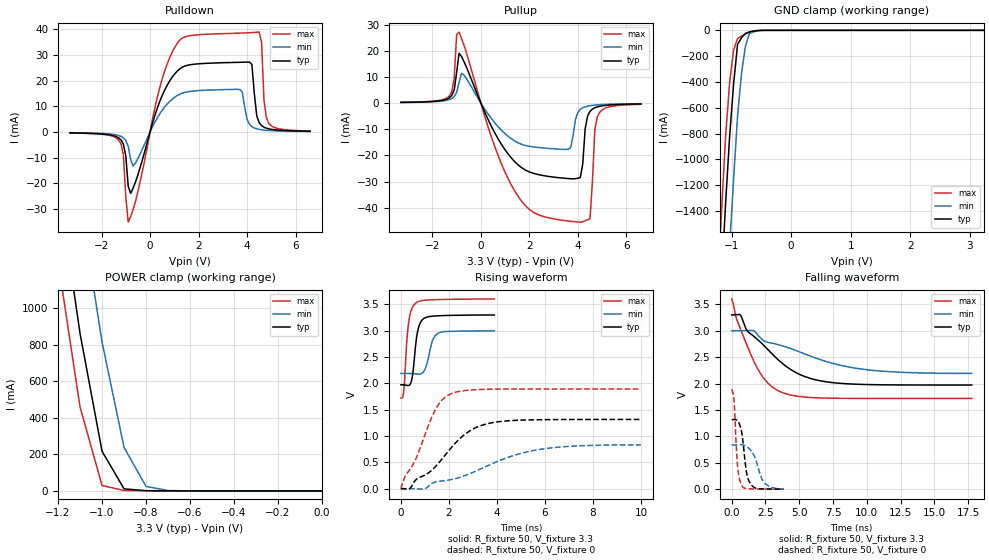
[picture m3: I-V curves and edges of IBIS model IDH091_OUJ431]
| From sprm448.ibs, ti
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|BUFFER IN NORMAL MODE WITHOUT PULLUP/PULLDOWN
|   Model Cell IDH091_OUJ431
|IDH091_OUJ431
[Model]   IDH091_OUJ431
Model_type   I/O
Polarity   Non-Inverting
Enable   Active-Low
Vinl =  0.8v
Vinh =  2v
Cref =  15.0000pF
Rref =  100.0000M
Vref =  0V
Vmeas =  1.65
C_comp   2.2553p   1.8929p   2.9061p
[Model Spec]
Vinl   0.8v   0.8v   0.8v
Vinh   2v   2v   2v
[Temperature Range]   25   125   -40
[Voltage Range]   3.3   3   3.6
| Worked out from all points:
|   slope of the pulldown table from 0 to 0.495 V, typ, clamps not added: 35.1 ohm
|   slope of the pullup table from 0 to 0.495 V, typ, clamps not added: 49.5 ohm
|   GND clamp passes 1 mA (typ) near -0.52 V on its own axis
|   POWER clamp passes 1 mA (typ) near -0.78 V on its own axis
|   rising waveform, R_fixture 50, V_fixture 3.3: 20-80 % time 211ps typ, 268ps min, 187ps max; typ from 1.97 V to 3.3 V
|   rising waveform, R_fixture 50, V_fixture 0: 20-80 % time 1.71ns typ, 2.93ns min, 1.06ns max; typ from 0 V to 1.31 V
|   falling waveform, R_fixture 50, V_fixture 3.3: 20-80 % time 3.49ns typ, 5.67ns min, 2.03ns max; typ from 3.3 V to 1.97 V
|   falling waveform, R_fixture 50, V_fixture 0: 20-80 % time 386ps typ, 697ps min, 250ps max; typ from 1.31 V to 0.002 V
[POWER_clamp]
|   voltage   I(typ)   I(min)   I(max)
-3.3V     22.03A     22.67A     21.68A
-1.2V     1.688A     2.438A     1.256A
-1.167V   1.413A     2.154A     990.6mA
-1.133V   1.137A     1.87A      725mA
-1.1V     861.3mA    1.585A     459.4mA
-1.033V   431.8mA    1.071A     173mA
-1V       217.1mA    814.3mA    29.74mA
-900mV    11.3mA     237.8mA    2.297mA
-800mV    1.149mA    24.8mA     1.228mA
-700mV    480.7uA    1.953mA    593.6uA
-11.55fV  74.41pA    10.75nA    861.5fA
[Pulldown]
|   voltage   I(typ)   I(min)   I(max)
-3.3V     -331.4uA   -255uA     -371.5uA
-1.3V     -2.223mA   -1.332mA   -3.045mA
-1.1V     -4.741mA   -2.234mA   -8.773mA
-900mV    -21.12mA   -5.605mA   -35.11mA
-700mV    -21.88mA   -13.27mA   -30.21mA
1.1V      23.53mA    14.08mA    34.28mA
3.7V      27.17mA    16.59mA    38.53mA
4.1V      27.25mA    2.984mA    38.69mA
4.5V      3.644mA    1.04mA     38.93mA
4.7V      1.881mA    774.1uA    12.24mA
4.9V      1.25mA     615uA      3.388mA
6.6V      316.3uA    220.9uA    418.1uA
[Pullup]
|   voltage   I(typ)   I(min)   I(max)
-3.3V     267.2uA    225.9uA    296.8uA
-1.3V     2.024mA    1.343mA    2.701mA
-900mV    19.01mA    7.852mA    27.16mA
500mV     -10.09mA   -6.71mA    -14.73mA
1.5V      -23.34mA   -15.02mA   -35.16mA
3.6V      -28.87mA   -17.67mA   -45.11mA
4.1V      -28.48mA   -2.422mA   -45.56mA
4.3V      -9.889mA   -1.421mA   -44.99mA
4.5V      -3.163mA   -993.4uA   -44.21mA
4.7V      -1.786mA   -760.3uA   -10.23mA
4.9V      -1.232mA   -614.5uA   -3.497mA
6.6V      -331.2uA   -231.1uA   -481.1uA
[GND_clamp]
|   voltage   I(typ)   I(min)   I(max)
-3.3V     -22.59A    -23.42A    -22.13A
-1.233V   -2.502A    -3.423A    -1.962A
-1.167V   -1.91A     -2.825A    -1.379A
-1.1V     -1.333A    -2.235A    -816.2mA
-1.033V   -822.7mA   -1.678A    -403.7mA
-966.7mV  -414.9mA   -1.154A    -152.8mA
-900mV    -109.4mA   -662.7mA   -63.5mA
-833.3mV  -56.6mA    -332.9mA   -43.85mA
-766.7mV  -24.29mA   -120.3mA   -26.9mA
-700mV    -12.46mA   -24.73mA   -12.65mA
-500mV    -344.8uA   -1.087mA   -120.5uA
3.233V    71.98pA    581.1nA    744.6fA
[Ramp]
| variable   typ   min   max
dV/dt_f  0.8025128/3.488897n   0.491601/5.741622n   1.136901/2.038879n
dV/dt_r  0.7945251/1.733254n   0.5072424/3.020166n   1.142074/1.063846n
R_load = 50
[Rising Waveform]
R_fixture = 50
V_fixture = 3.3
V_fixture_min = 3
V_fixture_max = 3.6
|   time   V(typ)   V(min)   V(max)
0s        1.972V     2.187V     1.718V
120ps     1.971V     2.188V     1.856V
248ps     1.962V     2.188V     2.797V
336ps     1.96V      2.187V     3.19V
464ps     2.092V     2.184V     3.423V
584ps     2.581V     2.18V      3.507V
744ps     3.071V     2.175V     3.553V
1.016ns   3.245V     2.278V     3.577V
1.544ns   3.282V     2.95V      3.589V
3.888ns   3.297V     2.994V     3.599V
[Rising Waveform]
R_fixture = 50
V_fixture = 0
V_fixture_min = 0
V_fixture_max = 0
|   time   V(typ)   V(min)   V(max)
0s        62.65pV    16.94nV    1.499pV
384ps     7.565mV    304.9uV    368.1mV
968ps     251.3mV    -3.495mV   980.9mV
1.384ns   392.9mV    119.5mV    1.454V
1.696ns   554.3mV    146.2mV    1.674V
2.072ns   764.9mV    170.5mV    1.798V
2.928ns   1.113V     296.4mV    1.874V
3.944ns   1.263V     502.7mV    1.89V
6.216ns   1.311V     772.1mV    1.893V
9.992ns   1.314V     831.5mV    1.893V
[Falling Waveform]
R_fixture = 50
V_fixture = 3.3
V_fixture_min = 3
V_fixture_max = 3.6
|   time   V(typ)   V(min)   V(max)
0s        3.3V       3V         3.6V
592ps     3.309V     3V         3.073V
1.152ns   2.998V     3.003V     2.713V
1.904ns   2.835V     2.931V     2.289V
2.688ns   2.641V     2.78V      2.007V
3.656ns   2.402V     2.72V      1.84V
5.36ns    2.138V     2.566V     1.746V
7.24ns    2.025V     2.399V     1.724V
11.2ns    1.977V     2.234V     1.718V
17.76ns   1.972V     2.193V     1.718V
[Falling Waveform]
R_fixture = 50
V_fixture = 0
V_fixture_min = 0
V_fixture_max = 0
|   time   V(typ)   V(min)   V(max)
0s        1.314V     837.5mV    1.893V
176ps     1.319V     838mV      1.664V
360ps     1.31V      840.2mV    707.1mV
448ps     1.29V      841.1mV    409.7mV
584ps     1.225V     842mV      188.3mV
752ps     1.06V      840mV      68.08mV
1.096ns   323.1mV    809.7mV    11.99mV
1.416ns   92.57mV    734mV      6.546mV
2.4ns     4.999mV    124.8mV    2.067mV
3.832ns   1.902mV    6.116mV    595.1uV
